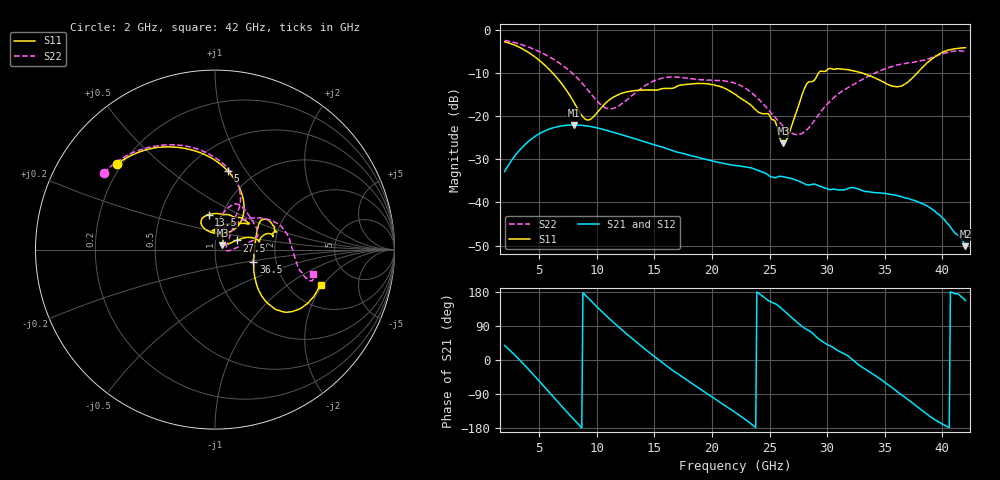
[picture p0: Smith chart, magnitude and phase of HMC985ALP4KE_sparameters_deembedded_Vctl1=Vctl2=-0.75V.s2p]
!s2p File: Measurements: S11, S21, S12, S22
# GHz S dB R 50.0
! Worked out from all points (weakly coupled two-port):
!   401 points, 2 GHz to 42 GHz, reference 50 ohm
!   highest |S21| = -22.05 dB at 8 GHz (marker M1); lowest = -50.1 dB at 42 GHz (marker M2)
!   lowest |S11| = -26.3 dB at 26.2 GHz (marker M3), VSWR 1.10, Z = 54.3 + j2.66 ohm
!   |S11| at or under -10 dB: 6.166 GHz to 29.26 GHz (23.09 GHz wide, 130 % of centre); 33.02 GHz to 37.82 GHz (4.802 GHz wide, 13.6 % of centre)
!   |S22| runs from -24.4 to -2.5 dB; largest |S21 - S12| = 0.00016
!   S11 on the Smith chart (normalised r, x): 2 GHz: 0.18, +0.36; 5 GHz: 0.76, +0.83; 13.5 GHz: 0.87, +0.35; 27.5 GHz: 1.27, +0.13; 36.5 GHz: 1.53, -0.21; 42 GHz: 2.97, -1.88
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2  -2.78 138.8  -32.87 38.2  -32.88 38.3  -2.47 145.3
3.4  -4.21 111.9  -27.61 -2.9  -27.62 -2.8  -3.38 122.8
5  -7.05 80.8  -24.10 -55.6  -24.11 -55.6  -5.05 98.1
6.3  -10.39 57.8  -22.65 -100.0  -22.65 -100.0  -6.93 79.8
8  -16.70 47.5  -22.05 -156.7  -22.06 -156.7  -10.36 62.2
8.7  -19.86 61.7  -22.14 -179.2  -22.15 -179.2  -12.30 58.8
9.5  -20.66 94.6  -22.44 155.9  -22.44 155.9  -14.83 59.1
11  -16.44 118.5  -23.41 111.7  -23.41 111.7  -18.31 74.6
13.5  -14.04 100.3  -25.41 45.7  -25.41 45.7  -14.28 79.2
15.4  -13.85 74.4  -26.96 0.1  -26.96 0.0  -11.41 68.3
18.9  -12.45 38.1  -29.66 -75.0  -29.67 -74.9  -11.54 40.8
22  -14.93 54.3  -31.43 -137.9  -31.44 -137.9  -12.39 16.0
24.9  -19.50 93.9  -33.69 156.8  -33.71 156.7  -18.54 4.7
26.2  -26.33 30.5  -34.07 131.0  -34.07 131.0  -22.41 -4.8
27.5  -17.69 23.1  -35.06 96.6  -35.03 96.6  -24.27 3.6
28.7  -11.99 10.4  -35.80 71.5  -35.79 71.5  -21.73 30.6
31  -9.03 21.1  -37.12 23.8  -37.13 23.8  -14.80 50.6
33.3  -10.26 32.4  -37.47 -23.8  -37.44 -23.9  -11.20 39.6
35.4  -12.79 11.1  -38.10 -67.8  -38.11 -67.8  -8.71 24.6
36.5  -13.01 -17.3  -38.72 -92.8  -38.75 -92.8  -7.90 15.8
39.6  -5.83 -42.6  -42.66 -162.0  -42.68 -161.7  -5.95 -15.5
42  -4.15 -18.3  -50.15 156.8  -50.13 155.0  -4.97 -14.0
